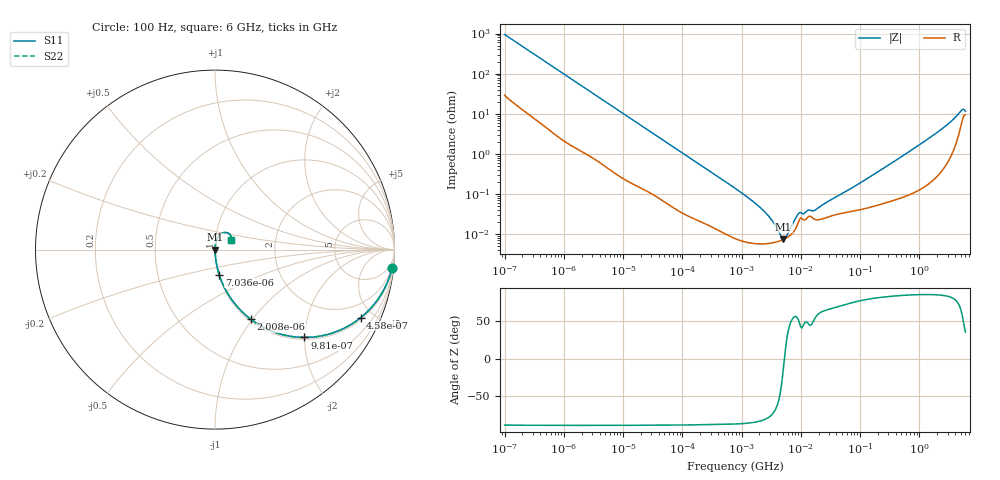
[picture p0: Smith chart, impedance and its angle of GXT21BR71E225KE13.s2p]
!Murata Part Number: GXT21BR71E225KE13
!These Parameters are Measured in Series Mode Connection
!Data Generated on Jan 08, 2026
!  o--ll--o
!Port1  Port2
!  o------o
!Operation Temp=25[degC], DC Bias Voltage=0[V]
!Freq. Start=100[Hz] Stop=6[GHz] 401[Steps]
# Hz S RI R 50
!Freq.(Hz) S11(Real) S11(Imag) S21(Real) S21(Imag) S12(Real) S12(Imag) S22(Real) S22(Imag)
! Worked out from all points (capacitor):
!   401 points, 100 Hz to 6 GHz, reference 50 ohm
!   read as one part in series: C = 1.67 uF near 109 Hz
!   lowest |Z| = 7.5 mohm at 5.079 MHz (marker M1)
!   series resonance near 5.283 MHz, so ESL is about 540 pH
!   S11 on the Smith chart (normalised r, x): 100 Hz: 2, -19; 458 Hz: 1.10, -4.23; 981 Hz: 1.04, -1.99; 2.008 kHz: 1.02, -0.98; 7.036 kHz: 1.01, -0.29; 6 GHz: 1.19, +0.13
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100  0.9859 -0.1036  0.0141 0.1036  0.0141 0.1036  0.9859 -0.1036
245  0.9335 -0.2366  0.0665 0.2366  0.0665 0.2366  0.9335 -0.2366
458  0.8115 -0.3794  0.1885 0.3794  0.1885 0.3794  0.8115 -0.3794
981  0.4984 -0.4894  0.5016 0.4894  0.5016 0.4894  0.4984 -0.4894
2008  0.1999 -0.3885  0.8001 0.3885  0.8001 0.3885  0.1999 -0.3885
3437  0.0828 -0.2637  0.9172 0.2637  0.9172 0.2637  0.0828 -0.2637
7036  0.0232 -0.1392  0.9768 0.1392  0.9768 0.1392  0.0232 -0.1392
40335  0.00143 -0.0256  0.9986 0.0256  0.9986 0.0256  0.00143 -0.0256
774597  7.87e-05 -0.00139  0.9999 0.00139  0.9999 0.00139  7.87e-05 -0.00139
2169299  5.68e-05 -0.000424  0.9999 0.000424  0.9999 0.000424  5.68e-05 -0.000424
3103719  5.91e-05 -0.000234  0.9999 0.000234  0.9999 0.000234  5.91e-05 -0.000234
4246196  6.59e-05 -9.32e-05  0.9999 9.32e-05  0.9999 9.32e-05  6.59e-05 -9.32e-05
5079039  7.31e-05 -1.68e-05  0.9999 1.68e-05  0.9999 1.68e-05  7.31e-05 -1.68e-05
6075234  8.47e-05 6.08e-05  0.9999 -6.08e-05  0.9999 -6.08e-05  8.47e-05 6.08e-05
9090158  0.000196 0.000254  0.9998 -0.000254  0.9998 -0.000254  0.000196 0.000254
1.360128e7  0.000274 0.000287  0.9997 -0.000287  0.9997 -0.000287  0.000274 0.000287
1.555665e7  0.000257 0.000277  0.9997 -0.000277  0.9997 -0.000277  0.000257 0.000277
1.779312e7  0.000228 0.000334  0.9998 -0.000334  0.9998 -0.000334  0.000228 0.000334
3.124326e8  0.000667 0.00537  0.9993 -0.00537  0.9993 -0.00537  0.000667 0.00537
2.142435e9  0.00437 0.0363  0.9956 -0.0363  0.9956 -0.0363  0.00437 0.0363
5.016141e9  0.0552 0.0957  0.9448 -0.0957  0.9448 -0.0957  0.0552 0.0957
6e9  0.0892 0.0562  0.9108 -0.0562  0.9108 -0.0562  0.0892 0.0562
